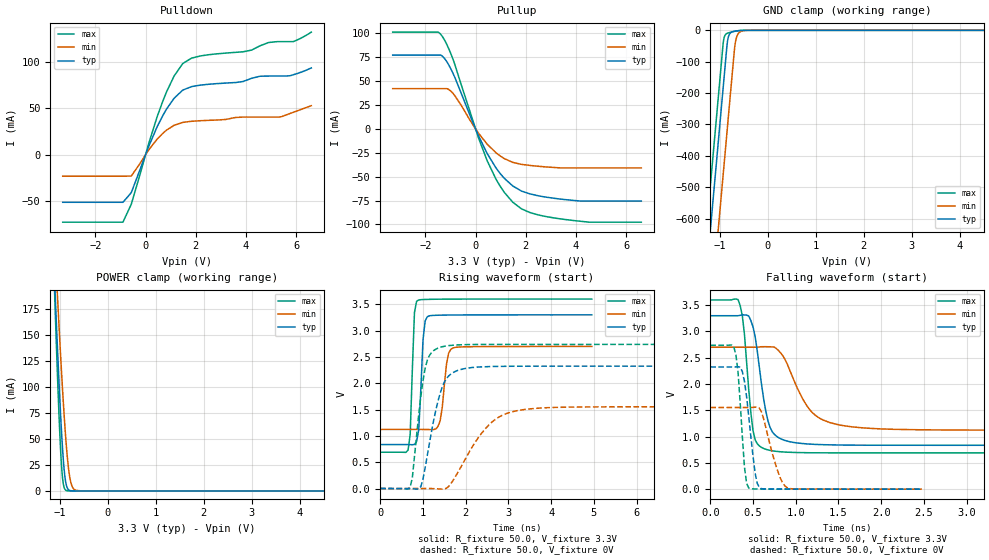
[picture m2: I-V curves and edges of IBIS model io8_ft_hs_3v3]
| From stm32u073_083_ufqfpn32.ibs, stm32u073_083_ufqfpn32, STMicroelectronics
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[Model]   io8_ft_hs_3v3
Model_type I/O
Polarity   Non-Inverting
Enable   Active-Low
| CAP_THRESHOLD on pad IOFT is "UDTCAPC" :
| Rising=30.0% of vddiom   Falling=70.0% of vddiom
| C_comp min and max val. don't necessarily correlate with the min and max pvt
| but are the smallest and greatest pad capacitance found.
| var   typ   min   max
C_comp   0.00000F  0.00000F  0.00000F
Vinl = 810.0mV
Vinh = 2.52V
Vmeas = 1.65V   | Reference voltage for timing measurements
Cref  = 50.0pF   | Timing specification test load capacitance value
Rref  = 100.0MOhm   | Timing specification test load resistance value
Vref  = 1.65V   | Timing specification test load voltage
[Model Spec]
| TIME_THRESHOLD on pin ZIV12 is "CMOS" :
| Rising=50.0% of vdd   Falling=50.0% of vdd
Vinl 1.34770V 1.11470V 1.44970V
Vinh 1.77530V 1.49030V 1.90330V
| variable   typ   min   max
[Temperature Range] 25.0 125.0 -40.0
| variable   typ   min   max
[Voltage Range] 3.3V 2.7V 3.6V
| variable   typ   min   max
[POWER Clamp Reference] 3.3V 2.7V 3.6V
| variable   typ   min   max
[GND Clamp Reference] 0V 0V 0V
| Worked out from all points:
|   slope of the pulldown table from 0 to 0.495 V, typ, clamps not added: 15.4 ohm
|   slope of the pullup table from 0 to 0.495 V, typ, clamps not added: 18.2 ohm
|   GND clamp passes 1 mA (typ) near -0.60 V on its own axis
|   POWER clamp passes 1 mA (typ) near -0.81 V on its own axis
|   rising waveform, R_fixture 50.0, V_fixture 3.3V: 20-80 % time 85.6ps typ, 124ps min, 75.1ps max; typ from 0.835 V to 3.3 V
|   falling waveform, R_fixture 50.0, V_fixture 3.3V: 20-80 % time 137ps typ, 308ps min, 93.5ps max; typ from 3.3 V to 0.835 V
|   rising waveform, R_fixture 50.0, V_fixture 0V: 20-80 % time 357ps typ, 767ps min, 238ps max; typ from 0 V to 2.33 V
|   falling waveform, R_fixture 50.0, V_fixture 0V: 20-80 % time 95.9ps typ, 158ps min, 68.1ps max; typ from 2.33 V to 0 V
[POWER Clamp]
-3.3V     2.991A     2.546A     3.694A
-1.11V    202.2mA    242.3mA    190.9mA
-1.09V    180mA      223.6mA    163.4mA
-1.05V    136.9mA    187mA      110.9mA
-1.01V    96.55mA    151.6mA    64.02mA
-970mV    60.39mA    117.9mA    27.41mA
-930mV    31.08mA    86.54mA    7.282mA
-860mV    4.779mA    40.5mA     315.2uA
-810mV    823.2uA    18.15mA    29.21uA
-760mV    129.2uA    6.282mA    2.687uA
-560mV    72.85nA    32.58uA    220.6pA
6.6V      0A         0A         0A
[GND Clamp]
-3.3V     -4.209A    -4.487A    -4.067A
-1.41V    -996.3mA   -1.274A    -854.3mA
-1.25V    -724.3mA   -1.002A    -582.3mA
-1.24V    -707.3mA   -984.6mA   -565.3mA
-940mV    -197.3mA   -474.6mA   -55.31mA
-930mV    -180.3mA   -457.6mA   -39.53mA
-840mV    -33.79mA   -304.6mA   -9.105mA
-790mV    -10.15mA   -219.6mA   -6.665mA
-680mV    -2.476mA   -41.57mA   -2.768mA
-630mV    -1.406mA   -13.77mA   -1.51mA
-530mV    -268.4uA   -1.762mA   -214.9uA
6.6V      833.9pA    196.4nA    597.5pA
| variable   typ   min   max
[Pullup Reference] 3.3V 2.7V 3.6V
| variable   typ   min   max
[Pulldown Reference] 0V 0V 0V
[Pullup]
-3.3V     77.35mA    42.24mA    101.4mA
-1.51V    77.35mA    42.24mA    101.4mA
-1.34V    76.54mA    42.24mA    97.42mA
-1.1V     68.45mA    41.76mA    85.85mA
-870mV    56.55mA    36.27mA    70.84mA
120mV     -7.358mA   -4.582mA   -9.588mA
460mV     -25.62mA   -15.84mA   -33.16mA
980mV     -46.64mA   -28.26mA   -59.98mA
1.48V     -59.67mA   -34.98mA   -76.65mA
2.17V     -68.03mA   -38.21mA   -87.55mA
3.19V     -72.79mA   -40.44mA   -93.41mA
6.6V      -75.45mA   -40.79mA   -97.6mA
[Pulldown]
-3.3V     -51.64mA   -23.39mA   -73.18mA
-900mV    -51.64mA   -23.39mA   -73.04mA
-570mV    -41.2mA    -23.23mA   -53.78mA
120mV     8.582mA    4.903mA    11.54mA
690mV     42.49mA    23.17mA    58.21mA
1.12V     60.48mA    31.51mA    84.25mA
1.48V     69.88mA    34.89mA    98.63mA
2.17V     75.22mA    36.71mA    106.8mA
3.88V     79.15mA    40.64mA    111.3mA
5.39V     85.07mA    40.9mA     122.4mA
5.88V     86.5mA     45.8mA     122.4mA
6.6V      93.9mA     53mA       132.7mA
[Ramp]
dV/dt_r 1.39485V/710.6362ps 931.93155mV/1.53332ns 1.64323V/471.61496ps
dV/dt_f 1.47909V/543.0213ps 946.45147mV/1.22574ns 1.74617V/364.2076ps
R_load = 50.0
| Removed startup time: 0s 0s 0s  .
| Removed end time: 4.95ns.
[Rising Waveform]
R_fixture   = 50.0
V_fixture   = 3.3V
V_fixture_min = 2.7V
V_fixture_max = 3.6V
0s        834.8mV    1.123V     689.8mV
650ps     834.5mV    1.123V     730.3mV
700ps     834.1mV    1.123V     1.027V
800ps     838.8mV    1.123V     3.345V
850ps     893.4mV    1.123V     3.558V
1ns       2.824V     1.122V     3.591V
1.1ns     3.264V     1.121V     3.594V
1.4ns     3.294V     1.284V     3.598V
1.7ns     3.297V     2.67V      3.599V
4.95ns    3.3V       2.7V       3.6V
| Removed startup time: 0s 0s 0s  .
| Removed end time: 4.975ns.
[Falling Waveform]
R_fixture   = 50.0
V_fixture   = 3.3V
V_fixture_min = 2.7V
V_fixture_max = 3.6V
0s        3.3V       2.7V       3.6V
325ps     3.3V       2.7V       3.608V
400ps     3.315V     2.7V       2.945V
500ps     3.087V     2.7V       1.115V
650ps     1.481V     2.711V     758.7mV
725ps     1.093V     2.707V     730.4mV
825ps     958.1mV    2.589V     710.9mV
1.15ns    858.6mV    1.542V     693.1mV
1.475ns   840.3mV    1.234V     690.4mV
4.975ns   834.9mV    1.123V     689.8mV
| Removed startup time: 0s 0s 0s  .
| Removed end time: 9.95ns.
[Rising Waveform]
R_fixture   = 50.0
V_fixture   = 0V
V_fixture_min = 0V
V_fixture_max = 0V
0s        -11.66uV   -15.19uV   -4.074uV
700ps     305.9uV    210.4nV    28.85mV
750ps     -1.922mV   715.8nV    202mV
950ps     37.18mV    31.86uV    1.754V
1.05ns    396.8mV    98.36uV    2.282V
1.4ns     1.807V     -10.85mV   2.683V
1.8ns     2.241V     283.8mV    2.729V
2.5ns     2.316V     1.173V     2.738V
3.15ns    2.324V     1.47V      2.739V
9.95ns    2.325V     1.553V     2.739V
| Removed startup time: 0s 0s 0s  .
| Removed end time: 2.475ns.
[Falling Waveform]
R_fixture   = 50.0
V_fixture   = 0V
V_fixture_min = 0V
V_fixture_max = 0V
0s        2.325V     1.553V     2.739V
275ps     2.325V     1.553V     2.711V
325ps     2.33V      1.553V     2.226V
375ps     2.237V     1.553V     1.005V
400ps     2.054V     1.553V     422.8mV
450ps     1.386V     1.553V     21.65mV
525ps     300.6mV    1.56V      3.581mV
600ps     9.714mV    1.466V     2.303mV
900ps     1.358mV    29.89mV    659.1uV
2.475ns   23.5uV     100.6uV    9.443uV
